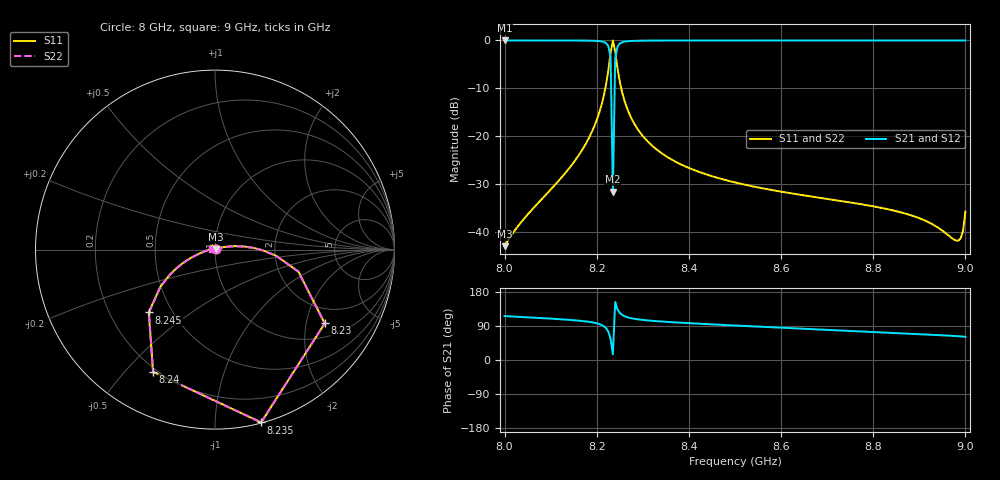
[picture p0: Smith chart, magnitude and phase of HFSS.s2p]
! Touchstone file from project
# GHZ S MA R 50.000000
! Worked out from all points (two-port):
!   201 points, 8 GHz to 9 GHz, reference 50 ohm
!   highest |S21| = -0.03 dB at 8 GHz (marker M1); lowest = -31.6 dB at 8.235 GHz (marker M2)
!   |S21| within 3 dB of the highest: start of sweep to 8.229 GHz; 8.242 GHz to end of sweep
!   lowest |S11| = -43.1 dB at 8 GHz (marker M3), VSWR 1.01, Z = 50.6 + j0.393 ohm
!   |S11| at or under -10 dB: start of sweep to 8.219 GHz; 8.253 GHz to end of sweep
!   |S22| runs from -43.1 to 0.0 dB; largest |S21 - S12| = 0
!   S11 on the Smith chart (normalised r, x): 8 GHz: 1.01, +0.01; 8.23 GHz: 1.43, -2.57; 8.235 GHz: 0.00, -1.30; 8.24 GHz: 0.18, -0.60; 8.245 GHz: 0.37, -0.35; 9 GHz: 0.98, +0.02
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8  0.007032 33.5  0.9971 115.9  0.9971 115.9  0.006979 23.5
! Gamma 8.777946E-002 2.295118E+002 8.782452E-002 2.295413E+002
! Port Impedance 5.000000E+001 0.000000E+000 5.000000E+001 0.000000E+000
8.17  0.07363 13.4  0.9944 102.7  0.9944 102.7  0.07363 12.6
8.2  0.1472 7.2  0.9862 96.8  0.9862 96.8  0.1472 6.8
8.22  0.3412 -5.6  0.9369 84.2  0.9369 84.2  0.3412 -5.8
8.225  0.4806 -14.7  0.8736 75.2  0.8736 75.2  0.4806 -14.8
8.23  0.7368 -33.9  0.6717 56.1  0.6717 56.1  0.7368 -33.9
8.235  0.9965 -75.1  0.02619 14.7  0.02619 14.7  0.9965 -75.0
8.24  0.7636 -116.9  0.6409 153.2  0.6409 153.2  0.7636 -116.8
8.245  0.5087 -136.5  0.8575 133.6  0.8575 133.6  0.5087 -136.4
8.255  0.2872 -151.1  0.9548 119.1  0.9548 119.1  0.2872 -150.9
8.275  0.1538 -160.2  0.9851 110.2  0.9851 110.2  0.1538 -159.8
8.3  0.09979 -164.8  0.9921 105.7  0.9921 105.7  0.09978 -164.2
8.335  0.06906 -168.7  0.9947 102.0  0.9947 102.0  0.06906 -167.9
8.405  0.04521 -174.2  0.996 96.9  0.996 96.9  0.0452 -173.0
8.5  0.03265 179.6  0.9965 91.0  0.9965 91.0  0.03263 -178.9
8.67  0.02309 169.4  0.9967 81.3  0.9967 81.3  0.02307 171.3
8.835  0.01699 159.5  0.9967 71.9  0.9967 71.9  0.01697 161.9
8.915  0.01285 154.2  0.9968 67.3  0.9968 67.3  0.01283 157.4
8.98  0.008037 145.7  0.9968 63.1  0.9968 63.1  0.007982 156.0
8.99  0.008523 142.6  0.9967 62.3  0.9967 62.3  0.008447 157.5
8.995  0.01023 140.8  0.9967 61.8  0.9967 61.8  0.01014 158.5
9  0.0162 138.8  0.9963 61.1  0.9963 61.1  0.01611 158.8
